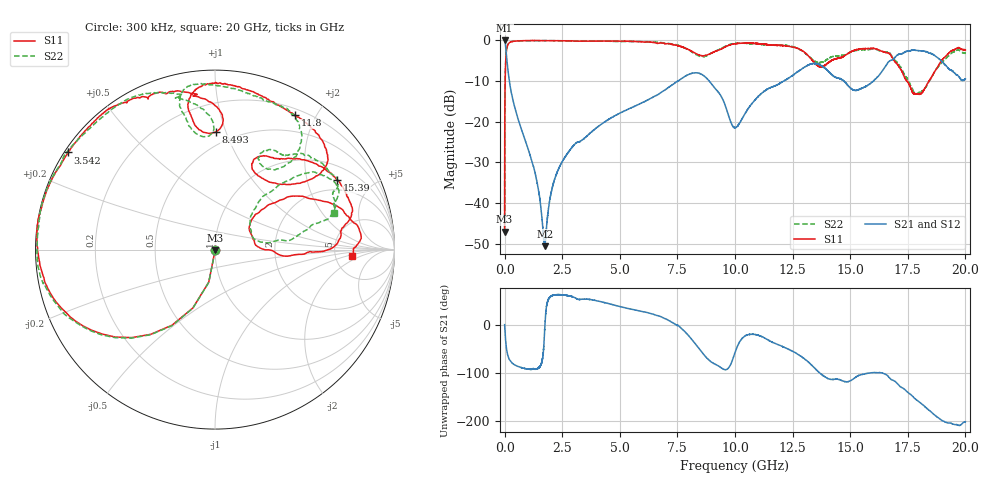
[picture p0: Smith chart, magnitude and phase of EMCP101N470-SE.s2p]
!EMCP101N470
!Johanson Technology Inc.
!www.johansontechnology.com
!Test Board Conditions:
!Substrate Type  RO4350B
!Substrate Thickness  10 mil
!Substrate Dk  3.66
!TL Type: GCPW
!TL Trace Width  20 mil
!TL Gap  10 mil
!PART MODE SINGLE ENDED (AKA BYPASS)
!DUT TOPOLOGY	SERIES-SHUNT
# MHz S  dB  R 50
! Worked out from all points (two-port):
!   20001 points, 300 kHz to 20 GHz, reference 50 ohm
!   highest |S21| = 0.01 dB at 300 kHz (marker M1); lowest = -50.6 dB at 1.745 GHz (marker M2)
!   |S21| within 3 dB of the highest: start of sweep to 69.87 MHz; 17.33 GHz to 18.4 GHz (1.062 GHz wide, 5.95 % of centre)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
!   lowest |S11| = -47.1 dB at 300 kHz (marker M3), VSWR 1.01, Z = 50 - j0.443 ohm
!   |S11| at or under -10 dB: start of sweep to 23.63 MHz; 17.47 GHz to 18.41 GHz (948.8 MHz wide, 5.29 % of centre); 18.41542 GHz to 18.41712 GHz (1.695 MHz wide, 0.00921 % of centre)
!   |S22| runs from -45.9 to 0.0 dB; largest |S21 - S12| = 0.017
!   S11 on the Smith chart (normalised r, x): 300 kHz: 1.00, -0.01; 3.542 GHz: 0.01, +0.30; 8.493 GHz: 0.40, +0.92; 11.8 GHz: 0.28, +1.72; 15.39 GHz: 1.54, +3.06; 20 GHz: 7.15, -1.32
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0.3  -47.05 -84.9  0.01 -0.2  -0.01 -0.2  -45.92 -80.9
102.298  -1.76 -146.4  -4.96 -55.9  -4.98 -55.9  -1.70 -146.3
164.298  -0.81 -158.3  -8.17 -67.6  -8.19 -67.6  -0.74 -158.2
524.292  -0.14 -178.2  -18.18 -85.3  -18.17 -85.5  -0.08 -175.2
1340.28  -0.02 170.4  -33.00 -91.9  -32.96 -91.9  -0.06 170.9
1745.274  -0.05 166.1  -50.60 -5.1  -50.21 -6.8  -0.03 165.0
2265.266  -0.05 161.3  -32.68 61.4  -32.66 61.5  -0.05 158.6
3334.25  -0.17 149.6  -24.63 52.3  -24.58 52.2  -0.14 150.3
3542.247  -0.15 146.6  -23.69 52.3  -23.64 52.4  -0.12 149.3
6667.2  -0.71 114.0  -13.27 18.3  -13.28 18.0  -0.44 113.7
8493.173  -3.68 89.7  -8.18 -53.0  -8.20 -53.0  -3.94 92.9
10000.15  -0.82 95.2  -21.47 -57.9  -21.42 -57.8  -0.72 99.5
11803.12  -1.20 59.3  -10.99 -40.2  -11.03 -40.4  -1.12 67.2
12671.11  -1.83 39.1  -7.86 -59.6  -7.94 -59.0  -1.79 53.6
13334.1  -4.73 39.3  -5.74 -84.1  -5.68 -83.9  -4.53 50.7
14055.09  -5.48 66.6  -7.61 -111.7  -7.48 -111.8  -4.47 64.4
15393.07  -2.13 29.7  -12.04 -104.7  -12.12 -105.6  -2.34 39.1
16667.05  -3.11 5.1  -5.20 -108.1  -5.20 -106.7  -2.85 20.7
17382.04  -9.34 -3.3  -2.81 -134.5  -2.78 -134.2  -8.69 8.3
18123.03  -12.79 34.0  -2.60 -164.5  -2.58 -164.5  -12.44 35.1
19331.01  -2.81 19.5  -7.19 156.9  -7.25 156.8  -3.44 39.5
20000  -2.36 -2.9  -9.47 159.5  -9.44 158.8  -3.23 16.6
